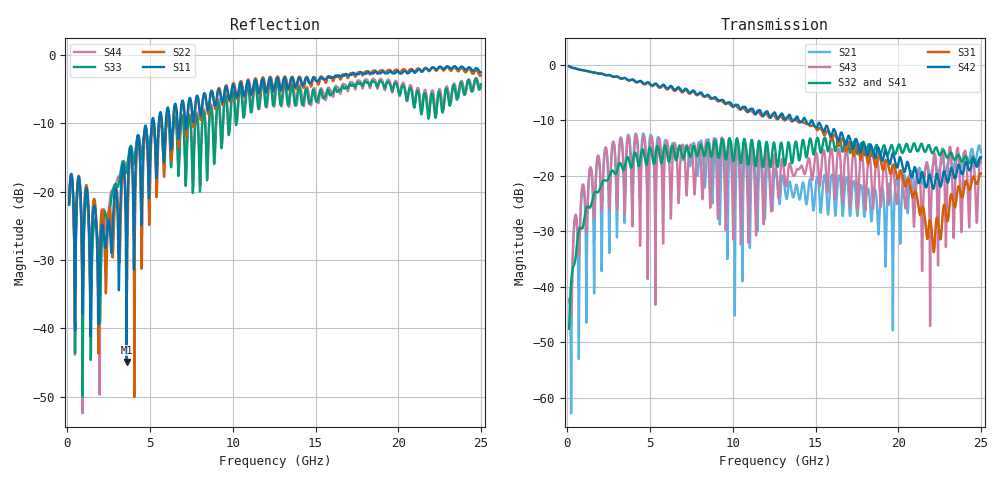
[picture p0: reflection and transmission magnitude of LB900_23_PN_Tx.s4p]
! Cadence S Parameter Output From FDA Version 1.0
! 4-dimension matrix file
# GHZ S RI R 50
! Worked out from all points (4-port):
!   2491 points, 100 MHz to 25 GHz, reference 50 ohm
!   strongest paths, dB at 100 MHz, 6.32 GHz, 12.55 GHz, 18.78 GHz, 25 GHz:
!     S42: -0.3, -4.0, -8.7, -14.9, -16.6
!     S31: -0.3, -4.2, -9.4, -16.6, -19.6
!     S32: -47.6, -14.6, -14.9, -15.2, -16.8
!     S41: -47.6, -14.8, -14.9, -15.4, -16.5
!     S43: -42.5, -19.6, -16.4, -17.9, -17.6
!     S21: -42.8, -14.4, -18.8, -29.8, -15.8
!   lowest |S11| = -44.9 dB at 3.57 GHz (marker M1), VSWR 1.01, Z = 50.6 + j0.122 ohm
!   |S11| at or under -10 dB: start of sweep to 5.104 GHz; 5.236 GHz to 5.52 GHz (284.5 MHz wide, 5.29 % of centre); 5.716 GHz to 5.946 GHz (230.9 MHz wide, 3.96 % of centre)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
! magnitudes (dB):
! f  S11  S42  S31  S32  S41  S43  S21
! 100 MHz  -21.7  -0.3  -0.3  -47.6  -47.6  -42.5  -42.8
! 1.93 GHz  -33.5  -1.6  -1.6  -22.6  -22.6  -17.4  -17.8
! 3.57 GHz  -44.9  -2.6  -2.6  -16.9  -17.2  -16.2  -15.1
! 6.51 GHz  -7.1  -4.6  -4.7  -16.7  -17.0  -14.2  -16.1
! 19.67 GHz  -2.7  -16.0  -18.1  -15.0  -15.1  -18.4  -44.3
! 22.13 GHz  -1.8  -22.3  -33.5  -15.8  -15.8  -17.2  -18.0
! 25 GHz  -2.5  -16.6  -19.6  -16.8  -16.5  -17.6  -15.8
